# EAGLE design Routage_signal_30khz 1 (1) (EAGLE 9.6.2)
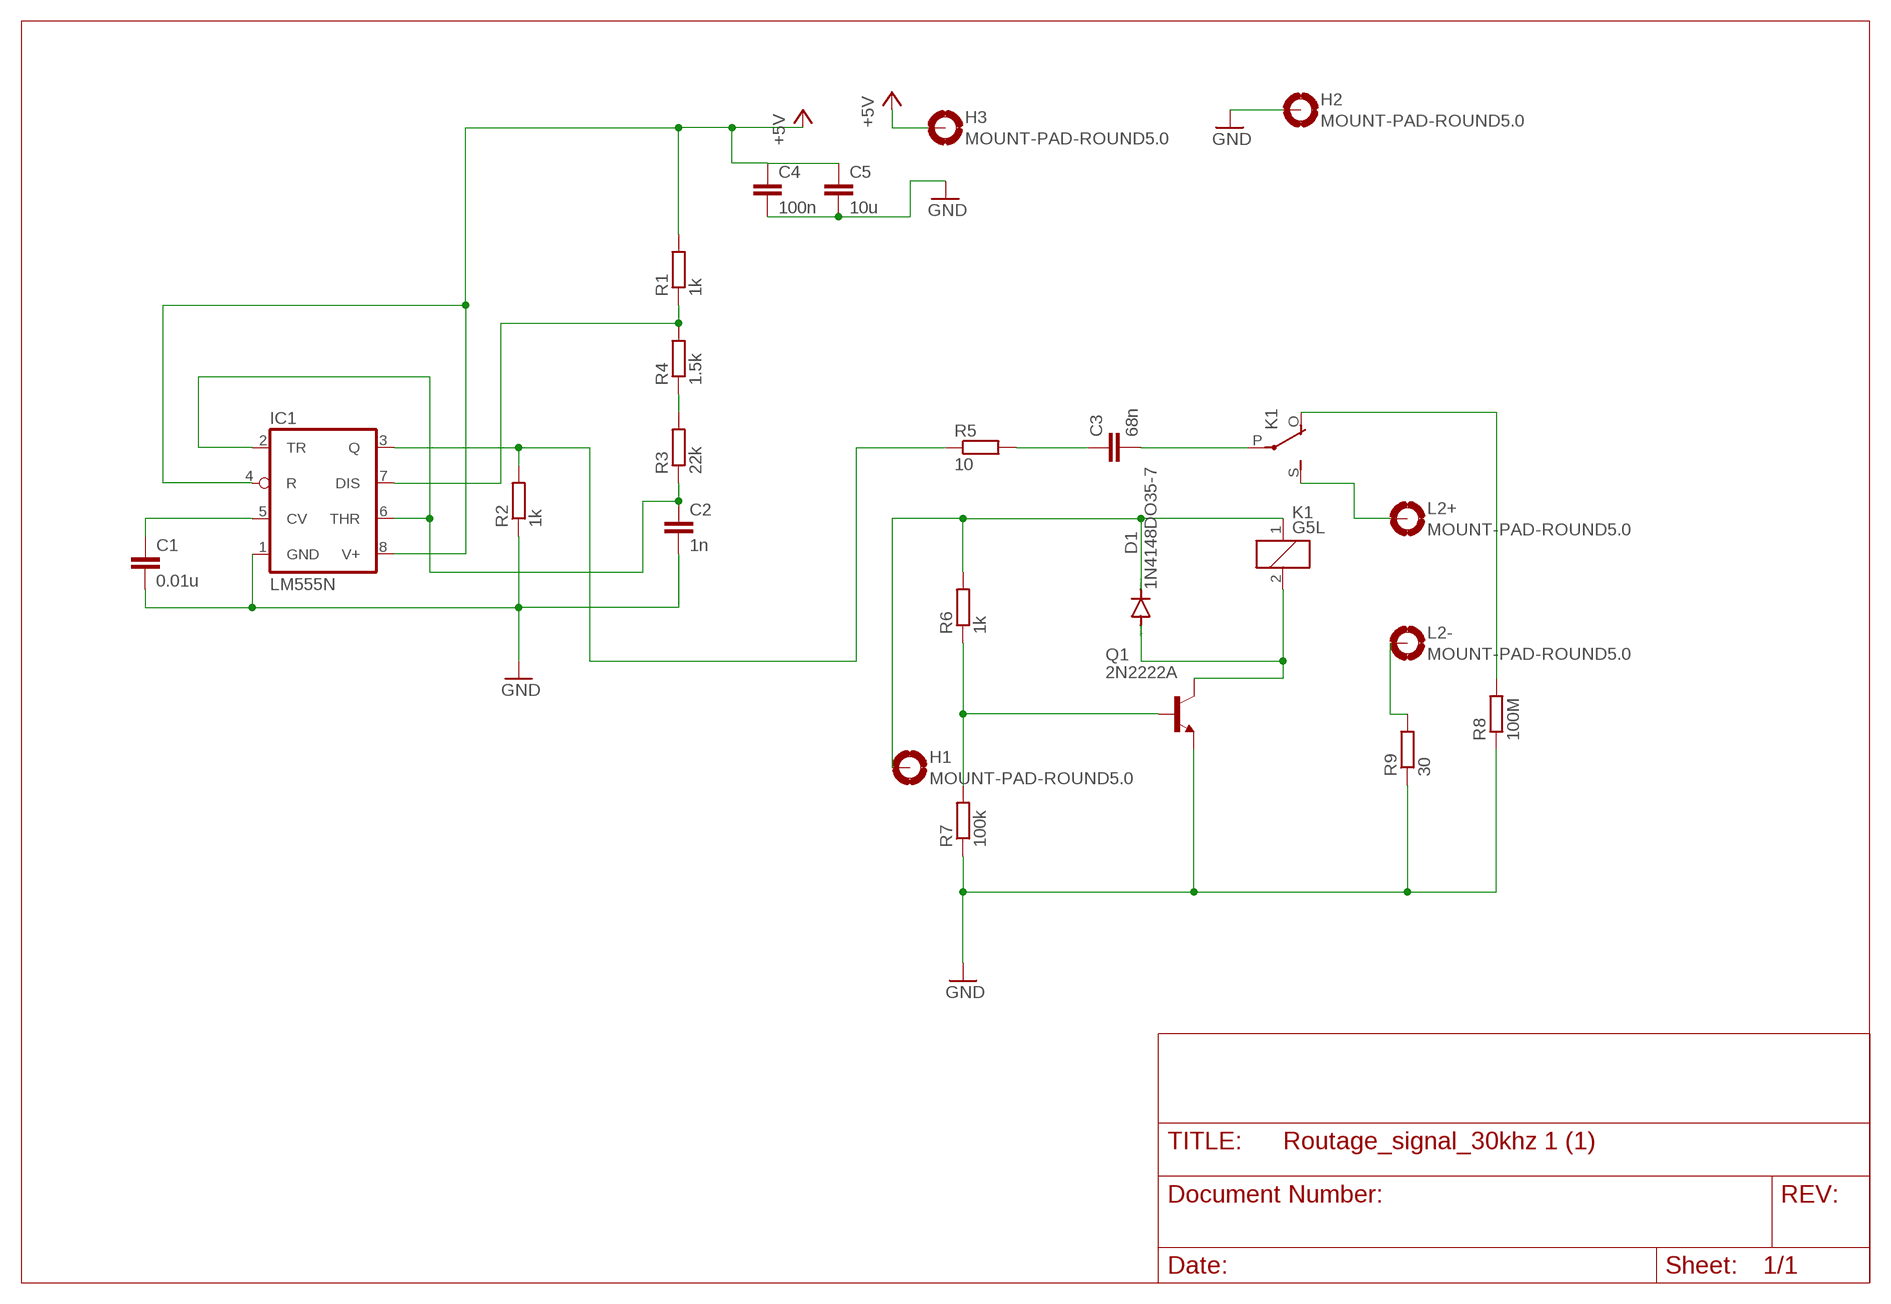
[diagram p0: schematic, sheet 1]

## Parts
C1  0.01u  C-EU025-025X050  [C025-025X050]
C2  1n  C-EU025-025X050  [C025-025X050]
C3  68n  C-EU025-025X050  [C025-025X050]
C4  100n  C-EU025-025X050  [C025-025X050]
C5  10u  C-EU025-025X050  [C025-025X050]
D1  1N4148DO35-7  [DO35-7]
H1  MOUNT-PAD-ROUND5.0  [5,0-PAD]
H2  MOUNT-PAD-ROUND5.0  [5,0-PAD]
H3  MOUNT-PAD-ROUND5.0  [5,0-PAD]
IC1  LM555N  [DIL08]
K1  G5L  [G5LE]
L2+  MOUNT-PAD-ROUND5.0  [5,0-PAD]
L2-  MOUNT-PAD-ROUND5.0  [5,0-PAD]
Q1  2N2222A  [TO18]
R1  1k  R-EU_0207/10  [0207/10]
R2  1k  R-EU_0207/10  [0207/10]
R3  22k  R-EU_0207/10  [0207/10]
R4  1.5k  R-EU_0207/10  [0207/10]
R5  10  R-EU_0207/10  [0207/10]
R6  1k  R-EU_0207/10  [0207/10]
R7  100k  R-EU_0207/10  [0207/10]
R8  100M  R-EU_0207/10  [0207/10]
R9  30  R-EU_0207/10  [0207/10]

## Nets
+5V: C4.1 C5.1 H3.B5(MOUNT) IC1.4(R) IC1.8(V+) R1.2
GND: C1.2 C2.2 C4.2 C5.2 H2.B5(MOUNT) IC1.1(GND) Q1.1(E) R2.1 R7.1 R8.1 R9.1
N$1: IC1.3(Q) R2.2 R5.1
N$2: C1.1 IC1.5(CV)
N$3: C2.1 IC1.2(TR) IC1.6(THR) R3.1
N$4: C3.1 R5.2
N$5: R3.2 R4.1
N$6: IC1.7(DIS) R1.1 R4.2
N$7: C3.2 K1.P(2:P)
N$8: K1.S(2:S) L2+.B5(MOUNT)
N$9: K1.O(2:O) R8.2
N$10: D1.C H1.B5(MOUNT) K1.1 R6.2
N$11: D1.A K1.2 Q1.3(C)
N$12: Q1.2(B) R6.1 R7.2
N$13: L2-.B5(MOUNT) R9.2

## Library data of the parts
C1-C5 = rcl:C-EU: CAPACITOR, European symbol; SPICEPREFIX: C
D1 = diode:1N4148: DIODE
H1-H3 L2+ L2- = holes:MOUNT-PAD-ROUND: MOUNTING PAD, round
IC1 = linear:*555: TIMER
K1 = relay:G5L: RELAY 1 x switch, 10 A/120 V AC, 8 A/30 V ADC, Omron; OC_FARNELL: unknown; OC_NEWARK: unknown
Q1 = transistor-npn:2N2222*: NPN Transistor
R1-R9 = rcl:R-EU_: RESISTOR, European symbol; SPICEPREFIX: R

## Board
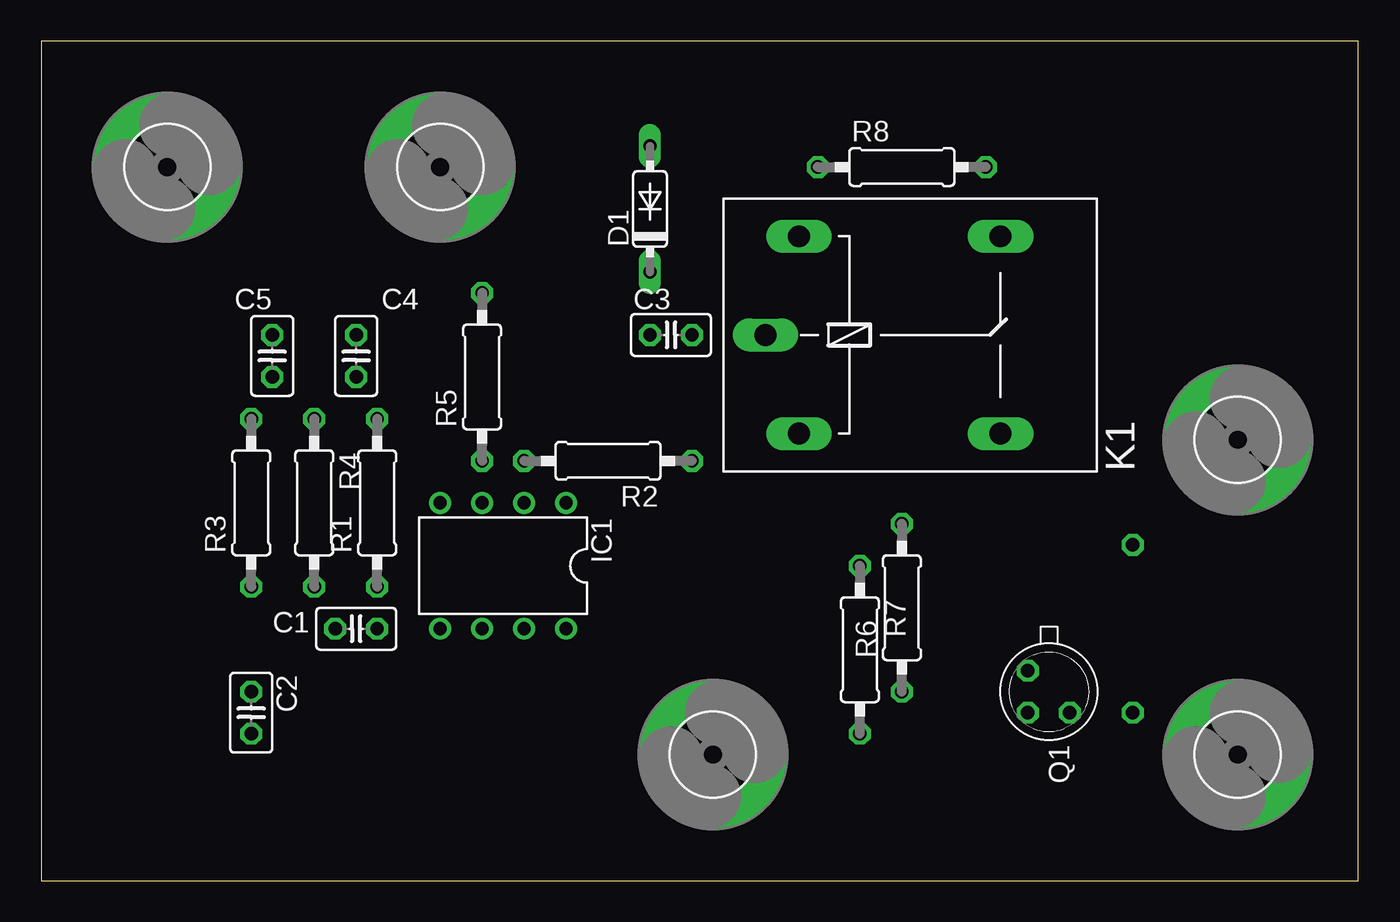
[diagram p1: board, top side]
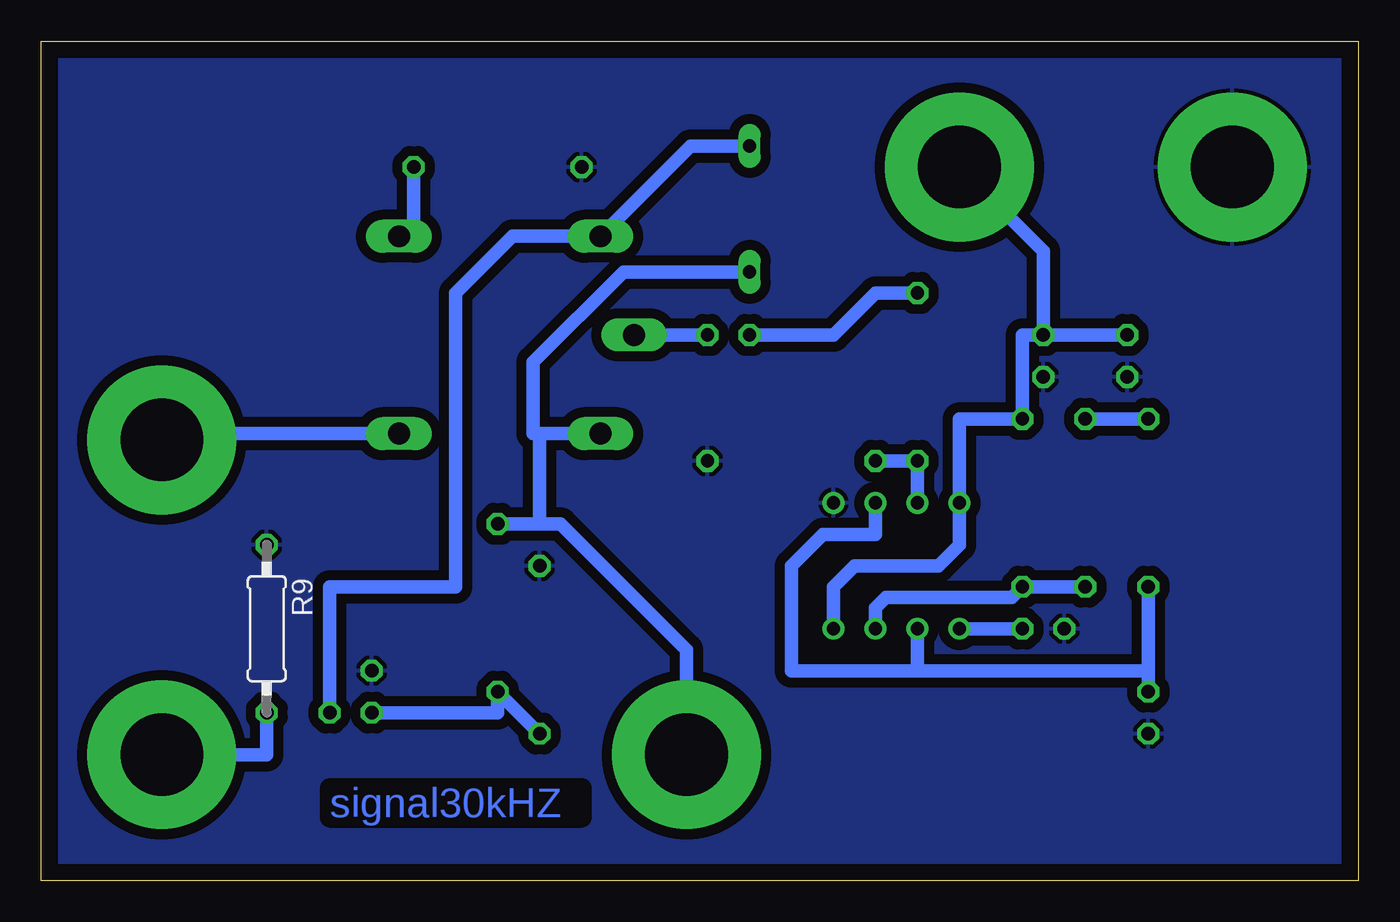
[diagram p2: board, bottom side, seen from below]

Size 79.68 x 50.79 mm. Coordinates in mm from the lower left corner, seen from the top.
Outline: 0,0 79.68,0 79.68,50.79 0,50.79 0,0
Copper layers (1*16): Top 0.035mm / dielectric 1.5mm / Bottom 0.035mm
Design rules "default": minimum track width 6mil, minimum drill 0.35mm, track to track 6mil, track to pad 6mil, pad to pad 6mil, via to via 6mil, smd to smd 6mil, copper to edge 40mil, drill to drill 6mil, minimum pad ring 10mil, minimum via ring 8mil, stop-mask expansion 4mil, vias tented up to drill 0mil, thermal gap 10mil

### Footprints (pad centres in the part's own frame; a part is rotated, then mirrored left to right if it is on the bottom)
C025-025X050 = drill 0.813 octagon: 1 -1.27,0; 2 1.27,0
DO35-7 = drill 0.813 long: A 3.81,0; C -3.81,0
5,0-PAD = drill 5 pad 9: B5 0,0
DIL08 = drill 0.813 pad 1.27: 1 -3.81,-3.81; 2 -1.27,-3.81; 3 1.27,-3.81; 4 3.81,-3.81; 5 3.81,3.81; 6 1.27,3.81; 7 -1.27,3.81; 8 -3.81,3.81
G5LE = drill 1.321 long: 1 -7.493,-5.969; 2 -7.493,5.969; O 4.699,5.969; P -9.525,0; S 4.699,-5.969
TO18 = drill 0.813 octagon: 1 -1.27,-1.27; 2 1.27,-1.27; 3 1.27,1.27
0207/10 = drill 0.813 octagon: 1 -5.08,0; 2 5.08,0

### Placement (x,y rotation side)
C1  19.05,15.24 180 top
C2  12.7,10.16 270 top
C3  38.1,33.02 0 top
C4  19.05,31.75 270 top
C5  13.97,31.75 270 top
D1  36.83,40.64 90 top
H1  40.64,7.62 0 top
H2  7.62,43.18 0 top
H3  24.13,43.18 0 top
IC1  27.94,19.05 180 top
K1  53.34,33.02 0 top
L2+  72.39,26.67 0 top
L2-  72.39,7.62 0 top
Q1  60.96,11.43 270 top
R1  20.32,22.86 90 top
R2  34.29,25.4 180 top
R3  12.7,22.86 90 top
R4  16.51,22.86 270 top
R5  26.67,30.48 90 top
R6  52.07,16.51 90 top
R7  49.53,13.97 270 top
R8  52.07,43.18 0 top
R9  66.04,15.24 270 bottom

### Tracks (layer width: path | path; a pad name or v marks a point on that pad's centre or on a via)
+5V
  Bottom 0.813: IC1.8 31.75,17.78 30.48,19.05 25.4,19.05 24.13,20.32 IC1.4 24.13,27.94 R1.2 20.32,33.02 C4.1 | C5.1 C4.1 | C4.1 19.05,38.1 H3.B5
GND
  pour Bottom (isolate 0.61): -1.27,81.28 101.6,81.28 101.6,-1.27 -1.27,-1.27
N$1
  Bottom 0.813: IC1.3 R5.1 R2.2
N$2
  Bottom 0.813: IC1.5 C1.1
N$3
  Bottom 0.813: IC1.6 26.67,12.7 | 26.67,12.7 34.29,12.7 34.29,19.05 32.38,20.95 29.21,20.95 IC1.2 | R3.1 12.7,12.7 | 12.7,12.7 C2.1 | 26.67,12.7 12.7,12.7
N$4
  Bottom 0.813: C3.1 31.75,33.02 29.21,35.56 R5.2
N$5
  Bottom 0.813: R4.1 R3.2
N$6
  Bottom 0.813: IC1.7 29.21,16.51 28.57,17.14 20.95,17.14 R1.1 R4.2
N$7
  Bottom 0.813: C3.2 K1.P
N$8
  Bottom 0.813: L2+.B5 72.01,27.05 K1.S
N$9
  Bottom 0.813: R8.2 57.15,39.88 K1.O
N$10
  Bottom 0.813: 49.53,21.59 48.26,21.59 40.64,13.97 H1.B5 | 49.53,21.59 R6.2 | 49.53,27.05 49.91,27.05 49.91,31.37 44.45,36.83 D1.C | 49.53,27.05 K1.1 | 49.53,27.05 49.53,21.59
N$11
  Bottom 0.813: Q1.3 62.23,17.78 54.61,17.78 54.61,35.56 51.18,38.99 K1.2 40.39,44.45 D1.A
N$12
  Bottom 0.813: R7.2 R6.1 52.07,10.16 Q1.2
N$13
  Bottom 0.813: L2-.B5 66.04,7.62 R9.2

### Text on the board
Bottom: signal30kHZ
